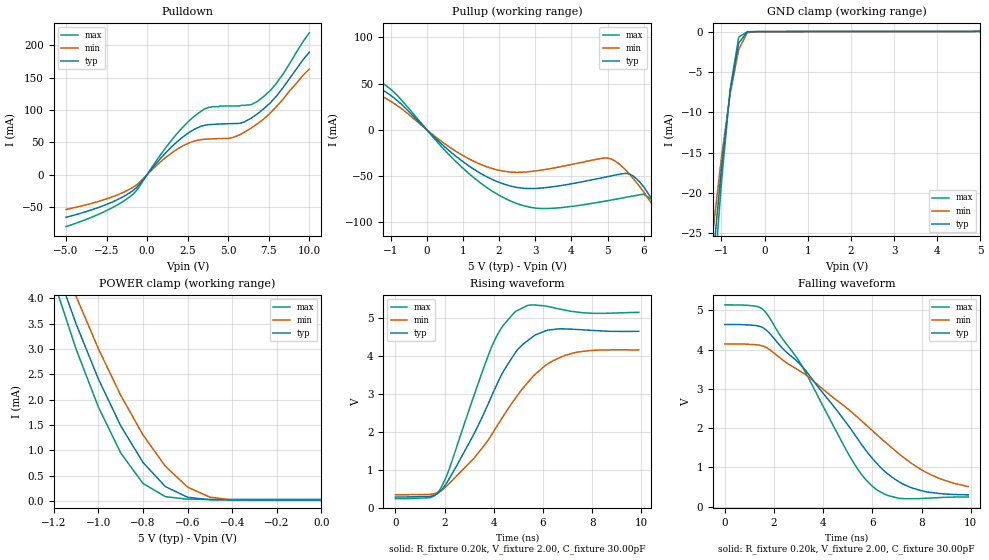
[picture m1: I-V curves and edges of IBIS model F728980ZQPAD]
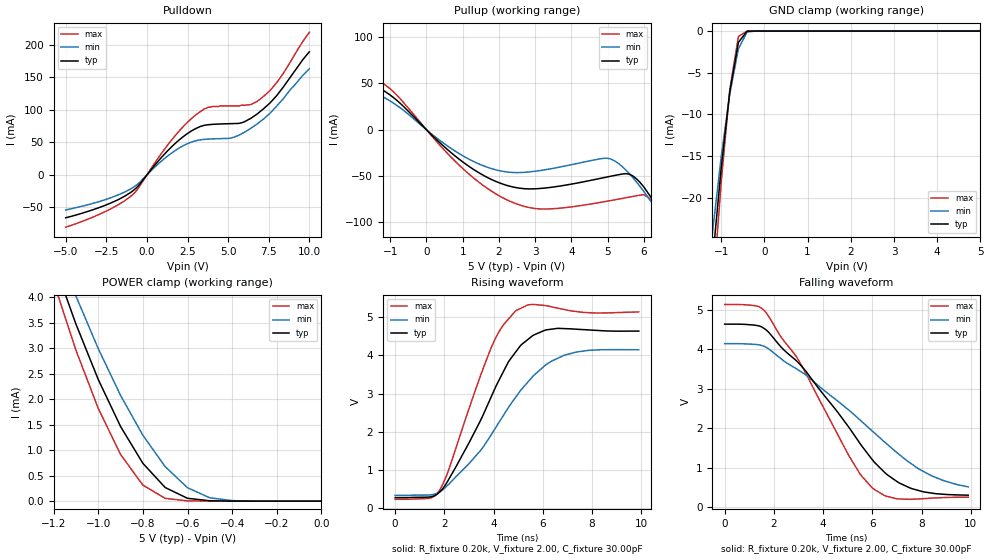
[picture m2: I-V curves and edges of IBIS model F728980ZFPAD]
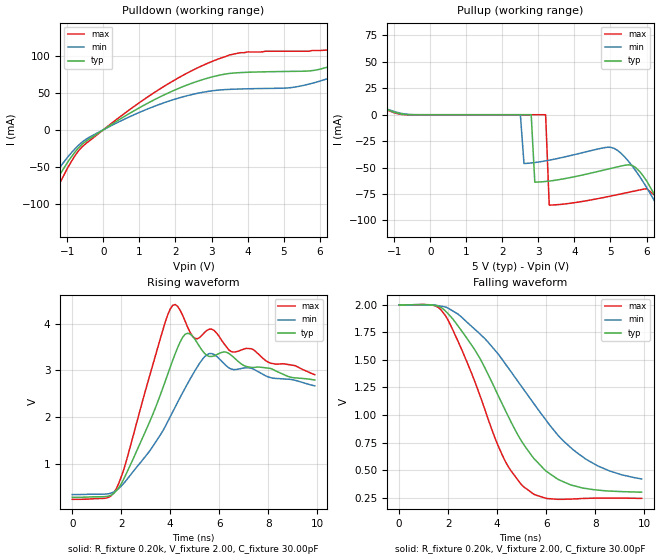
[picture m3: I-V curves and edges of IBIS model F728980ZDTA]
| IBIS file f728980.ibs created by s2ibis2 version 1.1
| North Carolina State University Electronics Research Laboratory  1995
[IBIS ver]   2.1
[File name]   f728980.ibs
[File Rev]   1.0
[Date]   02/03/2000
[Source]   Integrated Device Technology, Inc.
[Notes]   1. Temperatures: typ=25C, min=85C, max=-40C 2. Cemos9_5v
   process. 3. Ramp rates based on 50 ohm load.
[Copyright]   Copyright 1999, Integrated Device Technology, Inc.
|   Component idt728980z
[Component]   idt728980z
[Manufacturer]   Integrated Device Technology
[Package]
| variable   typ   min   max
R_pkg   0.75   0.60   0.90
L_pkg   8.10nH   8.30nH   9.90nH
C_pkg   0.53pF   0.46pF   0.60pF
[Pin]  signal_name   model_name   R_pin   L_pin   C_pin
1   DTA   F728980ZDTA
2   RX0   F728980ZTTL
3   RX1   F728980ZTTL
4   RX2   F728980ZTTL
5   RX3   F728980ZTTL
6   RX4   F728980ZTTL
7   RX5   F728980ZTTL
8   RX6   F728980ZTTL
9   RX7   F728980ZTTL
10   VCC   POWER
11   F0I   F728980ZTTL
12   C4I   F728980ZTTL
13   A0   F728980ZTTL
14   A1   F728980ZTTL
15   A2   F728980ZTTL
16   A3   F728980ZTTL
17   A4   F728980ZTTL
18   A5   F728980ZTTL
19   DS   F728980ZTTL
20   R_W   F728980ZTTL
21   CS   F728980ZTTL
22   D7   F728980ZQPAD
23   D6   F728980ZQPAD
24   D5   F728980ZQPAD
25   D4   F728980ZQPAD
26   D3   F728980ZQPAD
27   D2   F728980ZQPAD
28   D1   F728980ZQPAD
29   D0   F728980ZQPAD
30   GND   GND
31   TX7   F728980ZFPAD
32   TX6   F728980ZFPAD
33   TX5   F728980ZFPAD
34   TX4   F728980ZFPAD
35   TX3   F728980ZFPAD
36   TX2   F728980ZFPAD
37   TX1   F728980ZFPAD
38   TX0   F728980ZFPAD
39   ODE   F728980ZTTL
40   CCO   F728980ZFPAD
| Models and submodels in the file (4): F728980ZQPAD (I/O), F728980ZFPAD (3-state), F728980ZDTA (Output), F728980ZTTL (Input)
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| FIN  FIN   dummy_model
| FOEL FOEL   dummy_model
| QIN  QIN   dummy_model
| QOEL QOEL   dummy_model
| DIN  DIN   dummy_model
|   Model F728980ZQPAD
[Model]   F728980ZQPAD
Model_type   I/O
Polarity   Non-Inverting
Enable   Active-Low
Vinl =  0.000V
Vinh =  3.000V
Vmeas =  1.500V
C_comp   3.00pF   NA   NA
[Temperature Range]   25.00   85.00   -40.00
[Voltage Range]   5.00V   4.50V   5.50V
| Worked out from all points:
|   slope of the pulldown table from 0 to 0.75 V, typ, clamps not added: 33 ohm
|   slope of the pullup table from 0 to 0.75 V, typ, clamps not added: 27.8 ohm
|   GND clamp passes 1 mA (typ) near -0.54 V on its own axis
|   POWER clamp passes 1 mA (typ) near -0.83 V on its own axis
|   rising waveform, R_fixture 0.20k, V_fixture 2.00, C_fixture 30.00pF: 20-80 % time 2.03ns typ, 2.61ns min, 1.57ns max; typ from 0.28 V to 4.64 V
|   falling waveform, R_fixture 0.20k, V_fixture 2.00, C_fixture 30.00pF: 20-80 % time 3.27ns typ, 4.15ns min, 2.65ns max; typ from 4.64 V to 0.3 V
[Pulldown]
| voltage   I(typ)   I(min)   I(max)
-5V       -65.8mA    -53.7mA    -80.2mA
-2.6V     -47mA      -38.2mA    -56.7mA
-900mV    -25.12mA   -20mA      -30.8mA
1.7V      47.36mA    36.73mA    59.07mA
2.7V      66.85mA    50.03mA    85.52mA
3.5V      75.97mA    54.48mA    101mA
4V        77.55mA    55.27mA    105mA
5.3V      78.84mA    57.51mA    106mA
6V        81.62mA    65.55mA    107mA
6.8V      93.74mA    78.46mA    113mA
8V        122mA      106mA      142mA
10V       189mA      163mA      219mA
[Pullup]
| voltage   I(typ)   I(min)   I(max)
-5V       105mA      97.91mA    114mA
-3V       77.7mA     68.41mA    87.33mA
-1.4V     48mA       40.1mA     56.14mA
1V        -34.64mA   -28mA      -41.73mA
2.5V      -62.59mA   -46.24mA   -80.18mA
3.4V      -62.3mA    -42.33mA   -85.37mA
5V        -50.87mA   -30.79mA   -76.99mA
5.5V      -47.37mA   -43.73mA   -73.4mA
5.8V      -53.2mA    -57.29mA   -71.23mA
6.4V      -85.22mA   -90.13mA   -80.67mA
6.8V      -112mA     -114mA     -108mA
10V       -449mA     -401mA     -493mA
[GND_clamp]
| voltage   I(typ)   I(min)   I(max)
-5V       -304mA     -265mA     -346mA
-1.2V     -28.45mA   -24.98mA   -32.78mA
-1V       -17.04mA   -15.67mA   -18.78mA
-800mV    -7.561mA   -7.82mA    -7.246mA
-600mV    -1.42mA    -2.226mA   -692uA
-400mV    -29.13uA   -130uA     -8.943uA
-200mV    -2.063uA   -2.278uA   -3.142uA
5V        17.49uA    75.11uA    30.42uA
[POWER_clamp]
| voltage   I(typ)   I(min)   I(max)
-5V       75.88mA    69.99mA    82.76mA
-1.2V     4.719mA    5.164mA    4.333mA
-1.1V     3.493mA    4.035mA    2.995mA
-1V       2.405mA    3.003mA    1.851mA
-900mV    1.482mA    2.085mA    947uA
-800mV    759uA      1.302mA    345uA
-700mV    284uA      686uA      85.07uA
-600mV    73.03uA    273uA      35.57uA
-500mV    24.24uA    75.11uA    30.78uA
-400mV    18.03uA    20.22uA    30.51uA
0V        17.49uA    10.09uA    30.46uA
[Ramp]
| variable   typ   min   max
dV/dt_r   1.75/1.48n   1.36/2.44n   2.11/0.97n
dV/dt_f   1.61/3.90n   1.12/4.81n   2.03/3.08n
R_load = 50.00
[Rising Waveform]
R_fixture = 0.20k
V_fixture = 2.00
C_fixture = 30.00pF
R_dut = 0.75
L_dut = 8.10nH
C_dut = 0.53pF
| time   V(typ)   V(min)   V(max)
0s        280mV      338mV      236mV
1.4ns     297mV      351mV      265mV
1.8ns     421mV      423mV      463mV
2.1ns     667mV      578mV      864mV
3ns       1.706V     1.17V      2.583V
3.9ns     2.917V     1.907V     4.21V
4.9ns     4.102V     2.896V     5.168V
5.7ns     4.548V     3.517V     5.329V
6.9ns     4.702V     4.008V     5.196V
9.9ns     4.638V     4.15V      5.139V
[Falling Waveform]
R_fixture = 0.20k
V_fixture = 2.00
C_fixture = 30.00pF
R_dut = 0.75
L_dut = 8.10nH
C_dut = 0.53pF
| time   V(typ)   V(min)   V(max)
0s        4.642V     4.147V     5.141V
1.3ns     4.61V      4.124V     5.104V
1.7ns     4.49V      4.05V      4.919V
3.1ns     3.603V     3.436V     3.622V
5.2ns     1.907V     2.385V     1.155V
6.1ns     1.156V     1.876V     466mV
6.8ns     749mV      1.494V     257mV
7.6ns     479mV      1.099V     202mV
8.7ns     336mV      724mV      230mV
9.9ns     300mV      513mV      247mV
|   Model F728980ZFPAD
[Model]   F728980ZFPAD
Model_type   3-state
Polarity   Non-Inverting
Enable   Active-Low
Vinl =  0.000V
Vinh =  3.000V
Vmeas =  1.500V
C_comp   3.00pF   NA   NA
[Temperature Range]   25.00   85.00   -40.00
[Voltage Range]   5.00V   4.50V   5.50V
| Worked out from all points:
|   slope of the pulldown table from 0 to 0.75 V, typ, clamps not added: 33 ohm
|   slope of the pullup table from 0 to 0.75 V, typ, clamps not added: 27.8 ohm
|   GND clamp passes 1 mA (typ) near -0.55 V on its own axis
|   POWER clamp passes 1 mA (typ) near -0.84 V on its own axis
|   rising waveform, R_fixture 0.20k, V_fixture 2.00, C_fixture 30.00pF: 20-80 % time 2.02ns typ, 2.61ns min, 1.59ns max; typ from 0.28 V to 4.64 V
|   falling waveform, R_fixture 0.20k, V_fixture 2.00, C_fixture 30.00pF: 20-80 % time 3.24ns typ, 4.14ns min, 2.65ns max; typ from 4.64 V to 0.299 V
[Pulldown]
| voltage   I(typ)   I(min)   I(max)
-5V       -65.8mA    -53.8mA    -80.2mA
-2.6V     -47mA      -38.3mA    -56.7mA
-900mV    -25.13mA   -20mA      -30.8mA
1.7V      47.37mA    36.74mA    59.09mA
2.7V      66.87mA    50.04mA    85.55mA
3.5V      75.99mA    54.49mA    101mA
4V        77.57mA    55.28mA    105mA
5.3V      78.84mA    57.51mA    106mA
6V        81.62mA    65.55mA    107mA
6.8V      93.74mA    78.46mA    113mA
8V        122mA      106mA      142mA
10V       189mA      163mA      219mA
[Pullup]
| voltage   I(typ)   I(min)   I(max)
-5V       105mA      97.93mA    114mA
-3V       77.72mA    68.42mA    87.36mA
-1.4V     48.02mA    40.11mA    56.17mA
-800mV    31.1mA     25.71mA    36.62mA
1V        -34.64mA   -28mA      -41.73mA
2.5V      -62.59mA   -46.24mA   -80.18mA
3.4V      -62.3mA    -42.33mA   -85.37mA
5V        -50.87mA   -30.76mA   -76.99mA
5.8V      -52.96mA   -56.38mA   -71.23mA
6.4V      -84.1mA    -88.31mA   -80.31mA
6.8V      -110mA     -112mA     -107mA
10V       -441mA     -393mA     -486mA
[GND_clamp]
| voltage   I(typ)   I(min)   I(max)
-5V       -296mA     -257mA     -338mA
-1.2V     -27.64mA   -24.21mA   -31.93mA
-1V       -16.53mA   -15.17mA   -18.27mA
-800mV    -7.313mA   -7.552mA   -7.019mA
-600mV    -1.362mA   -2.139mA   -657uA
-400mV    -23.98uA   -122uA     -2.465uA
-200mV    -34.99nA   -915nA     -2.696nA
5V        50.36nA    65.06uA    50.29nA
[POWER_clamp]
| voltage   I(typ)   I(min)   I(max)
-5V       75.86mA    69.97mA    82.72mA
-1.2V     4.701mA    5.154mA    4.302mA
-1.1V     3.476mA    4.025mA    2.964mA
-1V       2.388mA    2.993mA    1.821mA
-900mV    1.465mA    2.075mA    917uA
-800mV    742uA      1.292mA    315uA
-700mV    267uA      676uA      54.61uA
-600mV    55.55uA    263uA      5.115uA
-500mV    6.778uA    65.06uA    331nA
-400mV    569nA      10.17uA    65.71nA
0V        50.36nA    49.98nA    55.34nA
[Ramp]
| variable   typ   min   max
dV/dt_r   1.75/1.46n   1.36/2.42n   2.11/0.94n
dV/dt_f   1.61/3.92n   1.12/4.82n   2.03/3.08n
R_load = 50.00
[Rising Waveform]
R_fixture = 0.20k
V_fixture = 2.00
C_fixture = 30.00pF
R_dut = 0.75
L_dut = 8.10nH
C_dut = 0.53pF
| time   V(typ)   V(min)   V(max)
0s        280mV      338mV      236mV
1.4ns     297mV      351mV      265mV
1.8ns     424mV      425mV      467mV
2.1ns     674mV      582mV      875mV
2.9ns     1.595V     1.105V     2.419V
3.9ns     2.914V     1.924V     4.204V
4.9ns     4.093V     2.91V      5.171V
5.6ns     4.525V     3.457V     5.334V
6.9ns     4.703V     4.012V     5.199V
9.9ns     4.638V     4.15V      5.139V
[Falling Waveform]
R_fixture = 0.20k
V_fixture = 2.00
C_fixture = 30.00pF
R_dut = 0.75
L_dut = 8.10nH
C_dut = 0.53pF
| time   V(typ)   V(min)   V(max)
0s        4.642V     4.147V     5.141V
1.3ns     4.609V     4.124V     5.103V
1.7ns     4.49V      4.049V     4.92V
3.3ns     3.447V     3.351V     3.389V
5ns       2.063V     2.482V     1.356V
6ns       1.2V       1.927V     482mV
6.6ns     821mV      1.595V     268mV
7.6ns     466mV      1.09V      195mV
8.5ns     343mV      768mV      227mV
9.9ns     299mV      508mV      247mV
|   Model F728980ZDTA
[Model]   F728980ZDTA
Model_type   Output
Vmeas =  1.500V
C_comp   3.00pF   NA   NA
[Temperature Range]   25.00   85.00   -40.00
[Voltage Range]   5.00V   4.50V   5.50V
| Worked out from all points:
|   slope of the pulldown table from 0 to 0.75 V, typ, clamps not added: 33 ohm
|   rising waveform, R_fixture 0.20k, V_fixture 2.00, C_fixture 30.00pF: 20-80 % time 1.26ns typ, 1.74ns min, 851ps max; typ from 0.28 V to 2.79 V
|   falling waveform, R_fixture 0.20k, V_fixture 2.00, C_fixture 30.00pF: 20-80 % time 2.5ns typ, 3.31ns min, 1.85ns max; typ from 2 V to 0.299 V
[Pulldown]
| voltage   I(typ)   I(min)   I(max)
-5V       -380mA     -327mA     -439mA
-2.6V     -177mA     -148mA     -209mA
-2.2V     -143mA     -119mA     -170mA
-1.8V     -109mA     -90.49mA   -130mA
-600mV    -20.02mA   -17.03mA   -23.44mA
1.4V      40.16mA    31.39mA    49.81mA
3.1V      72.32mA    53.05mA    93.85mA
5.7V      79.34mA    61.56mA    106mA
6.8V      93.74mA    78.46mA    113mA
8.4V      135mA      117mA      156mA
9.2V      163mA      141mA      189mA
10V       189mA      163mA      219mA
[Pullup]
| voltage   I(typ)   I(min)   I(max)
-5V       75.86mA    69.97mA    82.72mA
-1V       2.388mA    2.993mA    1.821mA
2.5V      25.05nA    21.9nA     30.07nA
2.6V      24.03nA    -46.16mA   29.06nA
2.8V      21.87nA    -45.62mA   27.03nA
2.9V      -63.8mA    -45.21mA   26.01nA
3.2V      -63.15mA   -43.62mA   22.66nA
3.3V      -62.75mA   -42.99mA   -85.48mA
5V        -50.87mA   -30.79mA   -76.99mA
5.6V      -47.95mA   -48.4mA    -72.67mA
6.8V      -114mA     -117mA     -109mA
10V       -460mA     -411mA     -504mA
[Ramp]
| variable   typ   min   max
dV/dt_r   0.69/0.55n   0.18/0.35n   1.23/0.54n
dV/dt_f   1.61/3.91n   1.12/4.83n   2.03/3.07n
R_load = 50.00
[Rising Waveform]
R_fixture = 0.20k
V_fixture = 2.00
C_fixture = 30.00pF
R_dut = 0.75
L_dut = 8.10nH
C_dut = 0.53pF
| time   V(typ)   V(min)   V(max)
0s        280mV      338mV      236mV
1.8ns     421mV      428mV      464mV
3.1ns     1.824V     1.23V      2.772V
4.1ns     3.211V     2.107V     4.388V
4.7ns     3.79V      2.706V     3.934V
5.1ns     3.587V     3.068V     3.671V
5.6ns     3.294V     3.358V     3.879V
6.5ns     3.317V     3.023V     3.398V
7.3ns     3.06V      3.045V     3.46V
9.9ns     2.79V      2.664V     2.905V
[Falling Waveform]
R_fixture = 0.20k
V_fixture = 2.00
C_fixture = 30.00pF
R_dut = 0.75
L_dut = 8.10nH
C_dut = 0.53pF
| time   V(typ)   V(min)   V(max)
0s        2V         2V         2V
1.4ns     1.997V     1.999V     1.995V
1.9ns     1.942V     1.98V      1.899V
3.1ns     1.587V     1.776V     1.297V
4.2ns     1.104V     1.506V     641mV
5.1ns     727mV      1.227V     345mV
6ns       490mV      952mV      243mV
7.3ns     348mV      651mV      239mV
8.6ns     309mV      491mV      246mV
9.9ns     299mV      419mV      243mV
